ORGANIZATION_BLOCK "Module Access Error"
TITLE =
VERSION : 0.1


VAR_TEMP
  OB122_EV_CLASS : BYTE ;	//16#29, Event class 2, Entering event state, Internal fault event
  OB122_SW_FLT : BYTE ;	//16#XX Software error code
  OB122_PRIORITY : BYTE ;	//X = Priority of OB where fault occured (Priority of 1 is lowest)
  OB122_OB_NUMBR : BYTE ;	//122 (Organization block 122, OB122)
  OB122_BLK_TYPE : BYTE ;	//16#88/8A/8C/8E Type of block fault occured in
  OB122_MEM_AREA : BYTE ;	//Memory area where access error occured
  OB122_MEM_ADDR : WORD ;	//Memory address where access error occured
  OB122_BLK_NUM : WORD ;	//Block number in which error occured
  OB122_PRG_ADDR : WORD ;	//Program address where error occured
  OB122_DATE_TIME : DATE_AND_TIME ;	//Date and time OB1 started
END_VAR
BEGIN
END_ORGANIZATION_BLOCK

